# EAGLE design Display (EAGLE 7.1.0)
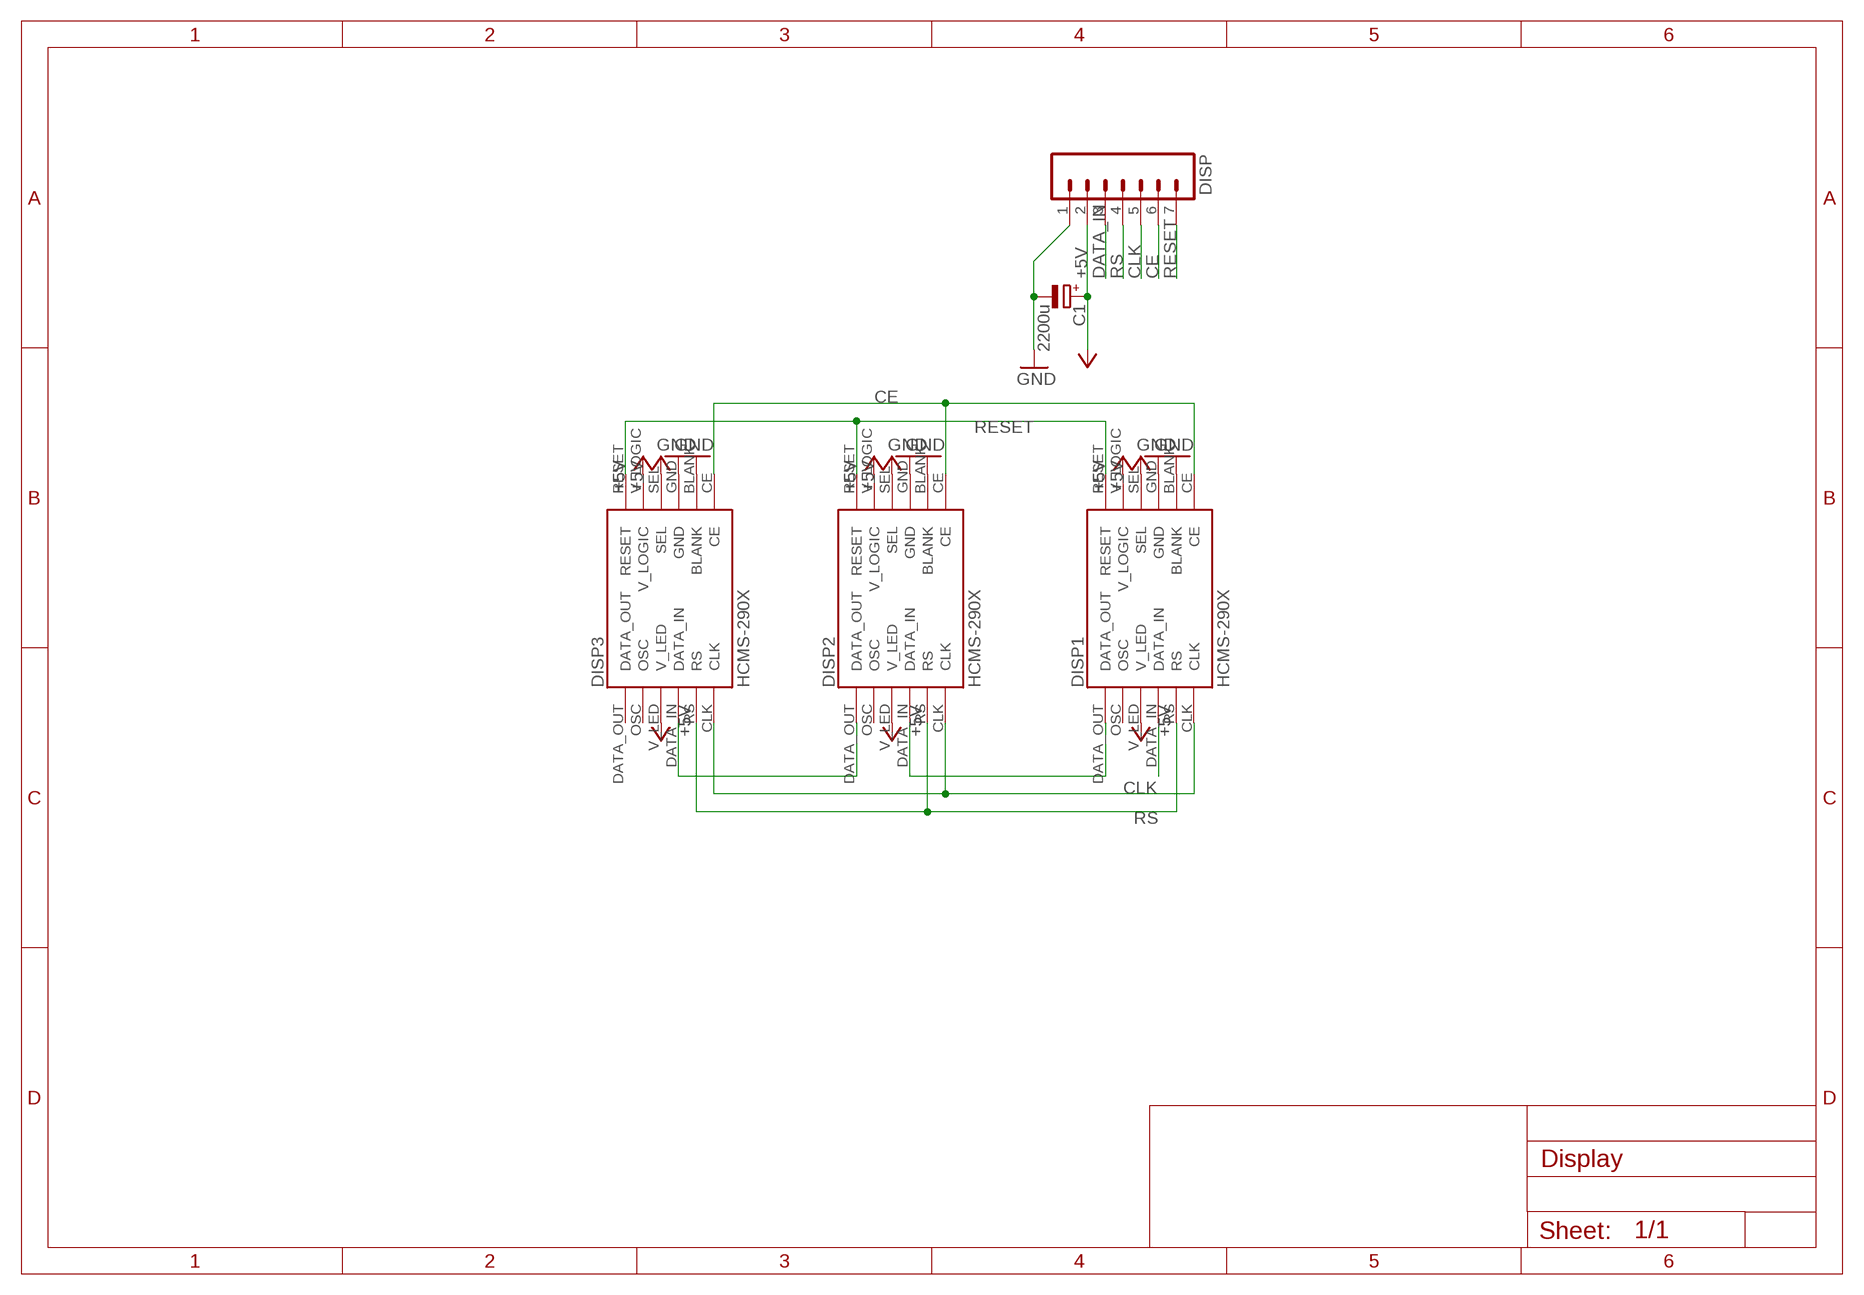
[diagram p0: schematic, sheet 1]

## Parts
C1  2200u  CPOL-EUE5-13  [E5-13]
DISP  M07  [1X07]
DISP1  HCMS-290X  [DIL6]
DISP2  HCMS-290X  [DIL6]
DISP3  HCMS-290X  [DIL6]

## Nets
+5V [Power]: C1.+ DISP1.SEL DISP1.V_LED DISP1.V_LOGIC DISP2.SEL DISP2.V_LED DISP2.V_LOGIC DISP3.SEL DISP3.V_LED DISP3.V_LOGIC DISP.2
CE: DISP1.CE DISP2.CE DISP3.CE DISP.6
CLK: DISP1.CLK DISP2.CLK DISP3.CLK DISP.5
DATA_IN: DISP1.DATA_IN DISP.3
DISP1-2: DISP1.DATA_OUT DISP2.DATA_IN
DISP2-3: DISP2.DATA_OUT DISP3.DATA_IN
GND [Ground]: C1.- DISP1.BLANK DISP1.GND DISP2.BLANK DISP2.GND DISP3.BLANK DISP3.GND DISP.1
RESET: DISP1.RESET DISP2.RESET DISP3.RESET DISP.7
RS: DISP1.RS DISP2.RS DISP3.RS DISP.4
Unconnected: DISP1.OSC DISP2.OSC DISP3.DATA_OUT DISP3.OSC

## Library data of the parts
C1 = rcl:CPOL-EU: POLARIZED CAPACITOR, European symbol
DISP = SparkFun-Connectors:M07: Header 7 Standard 7-pin 0.1" header. Use with straight break away headers (SKU : PRT-00116), right angle break away headers (PRT-00553), swiss pins (PRT-00743), machine pins (PRT-00117), and female headers (PRT-00115). NOTES ON THE VARIANTS LOCK and LOCK_LONGPADS... This footprint was designed to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
DISP1-DISP3 = avago-hcms-29xx:HCMS-290X

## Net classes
0 default: width 0.203 mm, drill 0.406 mm, clearance 0.203 mm
1 Power: width 0.61 mm, drill 0.711 mm, clearance 0.203 mm
2 Ground: width 0.508 mm, drill 0.711 mm, clearance 0.203 mm

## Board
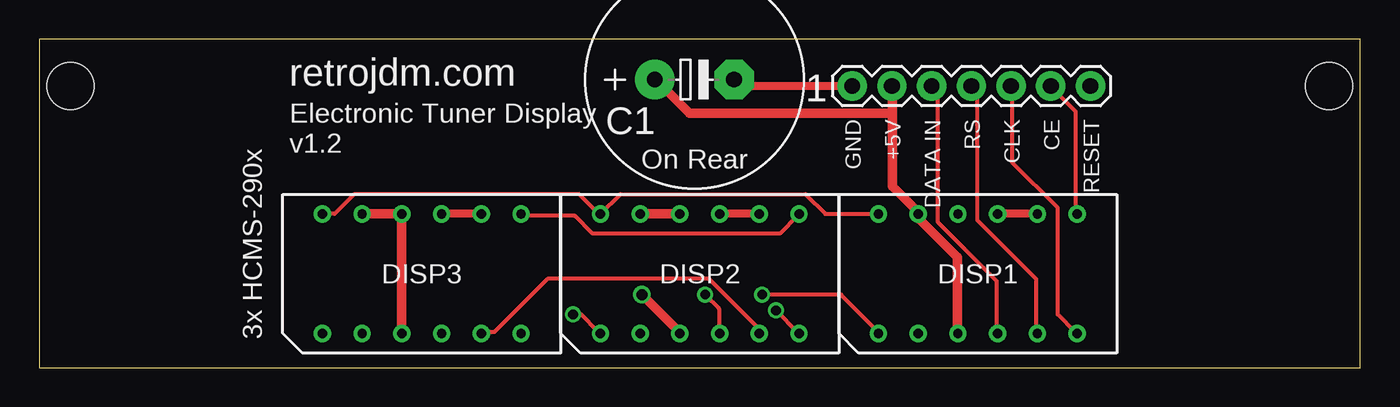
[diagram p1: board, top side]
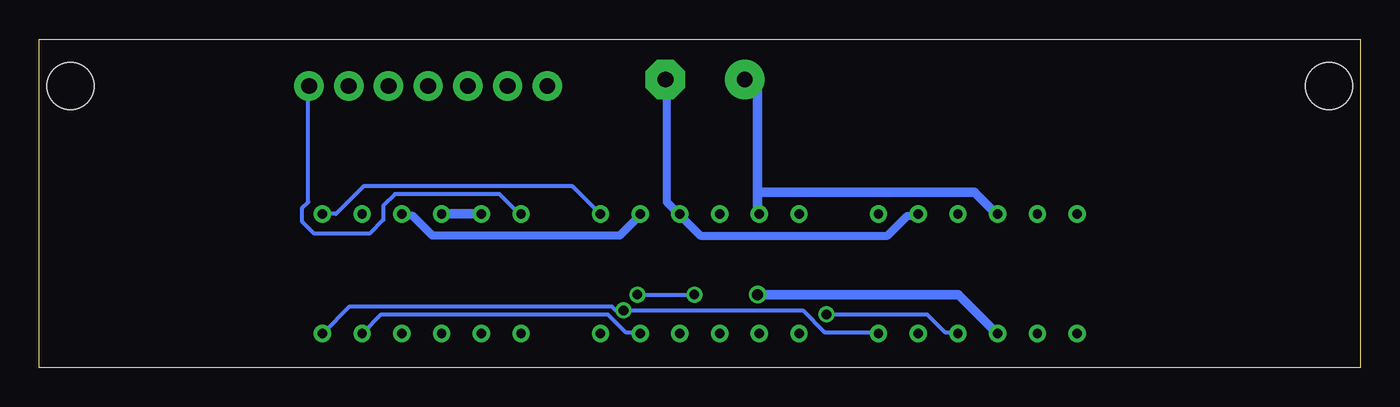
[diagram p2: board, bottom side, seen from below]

Size 84.5 x 21 mm. Coordinates in mm from the lower left corner, seen from the top.
Outline: 0,0 84.5,0 84.5,21 0,21 0,0
Copper layers (1*16): Top 0.035mm / dielectric 1.5mm / Bottom 0.035mm
Design rules "default *": minimum track width 10mil, minimum drill 24mil, track to track 0.25mm, track to pad 0.5mm, pad to pad 0.5mm, via to via 0.25mm, smd to smd 0.25mm, copper to edge 1mm, drill to drill 0.25mm, minimum pad ring 10mil, minimum via ring 8mil, stop-mask expansion 4mil, vias tented up to drill 0mil, thermal gap 10mil
Holes 3 mm at 2,18 82.5,18

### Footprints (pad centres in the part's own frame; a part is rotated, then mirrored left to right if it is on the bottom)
E5-13 = drill 1.016 pad 2.54: + -2.54,0 | drill 1.016 pad 2.54 octagon: - 2.54,0
1X07 = drill 1.016 pad 1.88: 1 0,0; 2 2.54,0; 3 5.08,0; 4 7.62,0; 5 10.16,0; 6 12.7,0; 7 15.24,0
DIL6 = drill 0.6: BLANK 3.81,3.81; CE 6.35,3.81; CLK 6.35,-3.81; DATA_IN 1.27,-3.81; DATA_OUT -6.35,-3.81; GND 1.27,3.81; OSC -3.81,-3.81; RESET -6.35,3.81; RS 3.81,-3.81; SEL -1.27,3.81; V_LED -1.27,-3.81; V_LOGIC -3.81,3.81

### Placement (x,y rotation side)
C1  41.91,18.41 0 top
DISP  52,18 0 top
DISP1  60.03,6 0 top
DISP2  42.25,6 0 top
DISP3  24.47,6 0 top

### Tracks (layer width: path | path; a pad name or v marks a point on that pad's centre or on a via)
+5V  (via drill 0.71)
  Top 0.61: DISP1.V_LED 58.72,2.27 58.72,7.06 56.32,9.45 56.32,9.7 DISP1.V_LOGIC 56.07,10.08 54.56,11.59 54.56,16.25 | 54.56,16.25 54.56,17.89 DISP.2 | DISP2.V_LOGIC 38.56,9.83 40.95,9.83 DISP2.SEL | DISP3.V_LOGIC 20.66,9.83 23.18,9.83 DISP3.SEL 23.18,9.58 23.18,2.27 DISP3.V_LED | v38.56,4.66 40.95,2.27 DISP2.V_LED | 54.56,16.25 41.58,16.25 39.44,18.4 C1.+
  Bottom 0.61: DISP1.V_LOGIC 56.32,9.83 58.72,9.83 DISP1.SEL | 38.56,11.21 38.56,17.64 39.31,18.4 C1.+ | 38.56,11.21 38.56,9.83 DISP2.V_LOGIC | v38.56,4.66 25.7,4.66 23.31,2.27 DISP3.V_LED | 38.56,11.21 24.7,11.21 23.31,9.83 DISP3.SEL
CE
  Top 0.254: DISP1.CE 66.28,9.83 66.28,16.38 64.76,17.89 DISP.6 | DISP3.CE 30.87,9.7 34.27,9.7 35.41,8.57 47.38,8.57 48.51,9.7 DISP2.CE
  Bottom 0.254: DISP1.CE 66.28,9.83 65.52,9.83 63.76,11.59 50.4,11.59 48.64,9.83 DISP2.CE
CLK  (via drill 0.61)
  Top 0.254: v47.12,3.65 48.51,2.27 DISP2.CLK | DISP.5 62.24,17.89 62.24,13.1 65.14,10.21 65.14,3.4 66.28,2.27 DISP1.CLK
  Bottom 0.254: DISP3.CLK 30.87,2.27 34.27,2.27 35.66,3.65 v47.12,3.65 47.63,3.65 47.88,3.91 64.64,3.91 66.28,2.27 DISP1.CLK
DATA_IN
  Top 0.254: DISP1.DATA_IN 61.24,2.27 61.24,5.54 57.46,9.32 57.46,17.64 57.2,17.89 DISP.3
DISP1-2  (via drill 0.61)
  Top 0.254: v42.59,4.66 43.47,3.78 43.47,2.27 DISP2.DATA_IN | v46.24,4.66 51.28,4.66 53.68,2.27 DISP1.DATA_OUT
  Bottom 0.254: v46.24,4.66 v42.59,4.66
DISP2-3  (via drill 0.61)
  Top 0.254: v34.15,3.4 34.65,3.4 35.78,2.27 DISP2.DATA_OUT
  Bottom 0.254: v34.15,3.4 27.72,3.4 26.59,2.27 25.83,2.27 DISP3.DATA_IN
GND
  Top 0.508: DISP.1 51.91,18.02 44.86,18.02 44.48,18.4 C1.- | DISP1.GND 61.36,9.83 63.76,9.83 DISP1.BLANK | DISP3.GND 25.83,9.83 28.22,9.83 DISP3.BLANK | DISP2.GND 43.6,9.83 45.99,9.83 DISP2.BLANK
  Bottom 0.508: DISP3.BLANK 28.35,9.7 28.98,9.7 30.24,8.44 42.21,8.44 43.47,9.7 DISP2.GND 43.72,9.95 44.35,10.58 44.35,18.4 C1.- | DISP1.GND 61.24,9.7 60.61,9.7 59.35,8.44 47.38,8.44 46.12,9.7 DISP2.BLANK
RESET
  Top 0.254: DISP3.RESET 18.14,9.83 18.9,9.83 20.16,11.09 34.52,11.09 35.78,9.83 DISP2.RESET 35.91,9.83 37.17,11.09 49.01,11.09 50.27,9.83 53.68,9.83 DISP1.RESET
  Bottom 0.254: DISP.7 67.28,17.89 67.28,10.58 67.66,10.21 67.66,9.32 66.91,8.57 63.38,8.57 62.5,9.45 62.5,10.33 61.74,11.09 55.06,11.09 53.8,9.83 DISP1.RESET
RS
  Top 0.254: DISP3.RS 28.35,2.27 29.11,2.27 32.51,5.67 42.84,5.67 45.99,2.52 45.99,2.27 DISP2.RS | DISP1.RS 63.76,2.27 63.76,5.67 59.98,9.45 59.98,17.64 59.72,17.89 DISP.4
  Bottom 0.254: DISP2.RS 46.12,2.27 47,2.27 48.13,3.4 62.62,3.4 63.76,2.27 DISP1.RS

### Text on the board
tNames: retrojdm.com | 1 | GND | +5V | DATA IN | RS | CLK | CE | RESET | 3x HCMS-290x | Electronic Tuner Display / v1.2 | On Rear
